FUNCTION_BLOCK FB_DO_IED_LD1_LPHD1_PhyNam EXTENDS FB_AcsiCommonDataClass
VAR_INPUT
	vendor: FB_AcsiDATypeVisString255 := (fc:=ACSI_FC_DC, sValue:='Beckhoff Automation', bLinkResult:=THIS^.AddDataToContainer(ipData:=vendor));
END_VAR
VAR
END_VAR

END_FUNCTION_BLOCK
